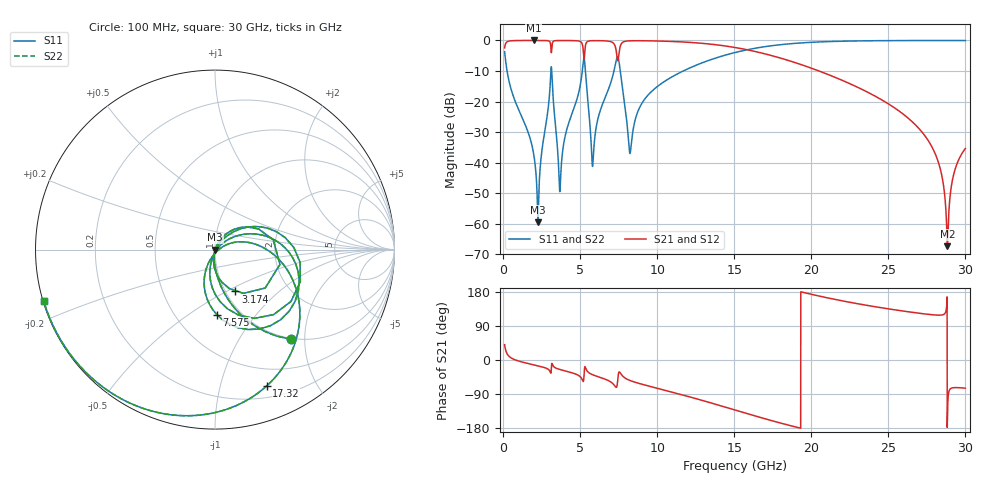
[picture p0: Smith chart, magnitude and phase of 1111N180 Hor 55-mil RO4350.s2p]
# GHz S MA R 50
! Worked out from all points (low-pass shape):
!   3201 points, 100 MHz to 30 GHz, reference 50 ohm
!   highest |S21| = -0.01 dB at 1.997 GHz (marker M1); lowest = -67.3 dB at 28.83 GHz (marker M2)
!   |S21| within 3 dB of the highest: start of sweep to 3.113 GHz; 7.555 GHz to 15.79 GHz (8.238 GHz wide, 70.6 % of centre)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
!   lowest |S11| = -59.5 dB at 2.258 GHz (marker M3), VSWR 1.00, Z = 50.1 - j0.0525 ohm
!   |S11| at or under -10 dB: 258.8 MHz to 3.105 GHz (2.846 GHz wide, 169 % of centre); 3.157 GHz to 5.141 GHz (1.984 GHz wide, 47.8 % of centre); 7.606 GHz to 11.69 GHz (4.082 GHz wide, 42.3 % of centre)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
!   |S22| runs from -59.5 to 0.0 dB; largest |S21 - S12| = 1e-11
!   S11 on the Smith chart (normalised r, x): 100 MHz: 0.98, -1.72; 3.174 GHz: 1.11, -0.55; 7.575 GHz: 0.78, -0.65; 17.32 GHz: 0.31, -1.40; 30 GHz: 0.00, -0.15
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0.1  0.656 -49.7  0.7545 40.3  0.7545 40.3  0.656 -49.7
1.996781  0.0133 -99.3  0.9988 -12.9  0.9988 -12.9  0.0133 -99.3
2.258406  0.001062 -29.6  0.9987 -15.4  0.9987 -15.4  0.001062 -29.6
3.174094  0.2591 -64.1  0.8275 -9.3  0.8275 -9.3  0.2591 -64.1
3.706688  0.004015 11.5  0.9964 -25.2  0.9964 -25.2  0.004015 11.5
5.089563  0.248 31.1  0.9237 -48.3  0.9237 -48.3  0.248 31.1
5.323156  0.361 -74.6  0.7533 -18.2  0.7533 -18.2  0.361 -74.6
5.837063  0.01047 0.1  0.9912 -39.3  0.9912 -39.3  0.01047 0.1
7.098469  0.2525 19.8  0.9288 -61.4  0.9288 -61.4  0.2525 19.8
7.575  0.3619 -88.4  0.751 -32.4  0.751 -32.4  0.3619 -88.4
8.24775  0.01433 -36.4  0.9854 -54.2  0.9854 -54.2  0.01433 -36.4
8.864437  0.08029 22.8  0.9889 -62.3  0.9889 -62.3  0.08029 22.8
10.06978  0.1809 13.3  0.9778 -75.3  0.9778 -75.3  0.1809 13.3
15.05  0.634 -42.5  0.7661 -132.0  0.7661 -132.0  0.634 -42.5
17.32053  0.8123 -69.2  0.5744 -158.8  0.5744 -158.8  0.8123 -69.2
20.03956  0.9324 -97.4  0.3491 173.0  0.3491 173.0  0.9324 -97.4
25.01978  0.9924 -135.7  0.09111 134.8  0.09111 134.8  0.9924 -135.7
27.86028  0.9965 -152.4  0.0175 119.4  0.0175 119.4  0.9965 -152.4
28.43959  0.9967 -155.4  0.006699 118.6  0.006699 118.6  0.9967 -155.4
28.83203  0.9967 -157.5  0.0004308 -158.6  0.0004308 -158.6  0.9967 -157.5
29.27119  0.9967 -159.7  0.006897 -72.9  0.006897 -72.9  0.9967 -159.7
30  0.9965 -163.3  0.01711 -74.4  0.01711 -74.4  0.9965 -163.3
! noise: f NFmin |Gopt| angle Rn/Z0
0.1  0.0006796  0.743  2.94  0.0005303
3.417  0.02147  0.7239  23.3  0.01482
6.743  0.03662  0.6948  44.15  0.02021
10.06  0.02955  0.5133  62.33  0.008039
13.39  0.03669  0.51  75.96  0.008605
16.7  0.05424  0.6031  90.83  0.01321
20.03  0.09178  0.7356  108.5  0.02474
23.35  0.1906  0.863  127.6  0.05943
26.67  0.6538  0.9579  146.3  0.2971
30  1.667  0.9828  163.2  0.4831
